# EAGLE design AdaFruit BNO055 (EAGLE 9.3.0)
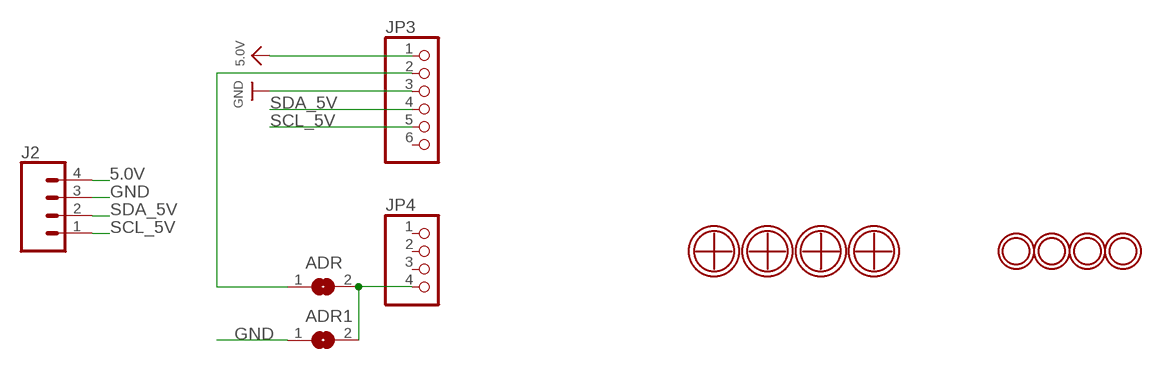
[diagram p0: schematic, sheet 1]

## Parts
ADR  SOLDERJUMPERREFLOW  [SOLDERJUMPER_REFLOW]
ADR1  SOLDERJUMPERREFLOW  [SOLDERJUMPER_REFLOW]
J2  CONN_04  [1X04]
JP3  HEADER-1X676MIL  [1X06_ROUND_76]
JP4  HEADER-1X476MIL  [1X04_ROUND_76]
U$1  3.2MM-5MM  [3.2MM-5MM]
U$3  3.2MM-5MM  [3.2MM-5MM]
U$4  3.2MM-5MM  [3.2MM-5MM]
U$5  3.2MM-5MM  [3.2MM-5MM]
U$7  MOUNTINGHOLE2.5_THICK  [MOUNTINGHOLE_2.5_PLATED_THICK]
U$8  MOUNTINGHOLE2.5_THICK  [MOUNTINGHOLE_2.5_PLATED_THICK]
U$9  MOUNTINGHOLE2.5_THICK  [MOUNTINGHOLE_2.5_PLATED_THICK]
U$11  MOUNTINGHOLE2.5_THICK  [MOUNTINGHOLE_2.5_PLATED_THICK]

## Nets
5.0V: J2.4 JP3.1
GND: ADR1.1 J2.3 JP3.3
N$1: ADR1.2 ADR.2 JP4.4
N$2: ADR.1 JP3.2
SCL_5V: J2.1 JP3.5
SDA_5V: J2.2 JP3.4
Unconnected: JP3.6 JP4.1 JP4.2 JP4.3 U$1.P$1 U$3.P$1 U$4.P$1 U$5.P$1

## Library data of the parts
ADR ADR1 = #microbuilder:SOLDERJUMPER: SMD Solder JUMPER
J2 = SparkFun-Connectors:CONN_04: Multi connection point. Often used as Generic Header-pin footprint for 0.1 inch spaced/style header connections On any of the 0.1 inch spaced packages, you can populate with these: Break Away Headers - Straight (PRT-00116) Break Away Male Headers - Right Angle (PRT-00553) Female Headers (PRT-00115)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; PROD_ID: CONN-09696
JP3 = microbuilder:HEADER-1X6: PIN HEADER
JP4 = microbuilder:HEADER-1X4: PIN HEADER
U$1 U$3-U$5 = #Holes:3.2MM-5MM
U$7-U$9 U$11 = microbuilder:MOUNTINGHOLE: Mounting Hole; BOM: EXCLUDE

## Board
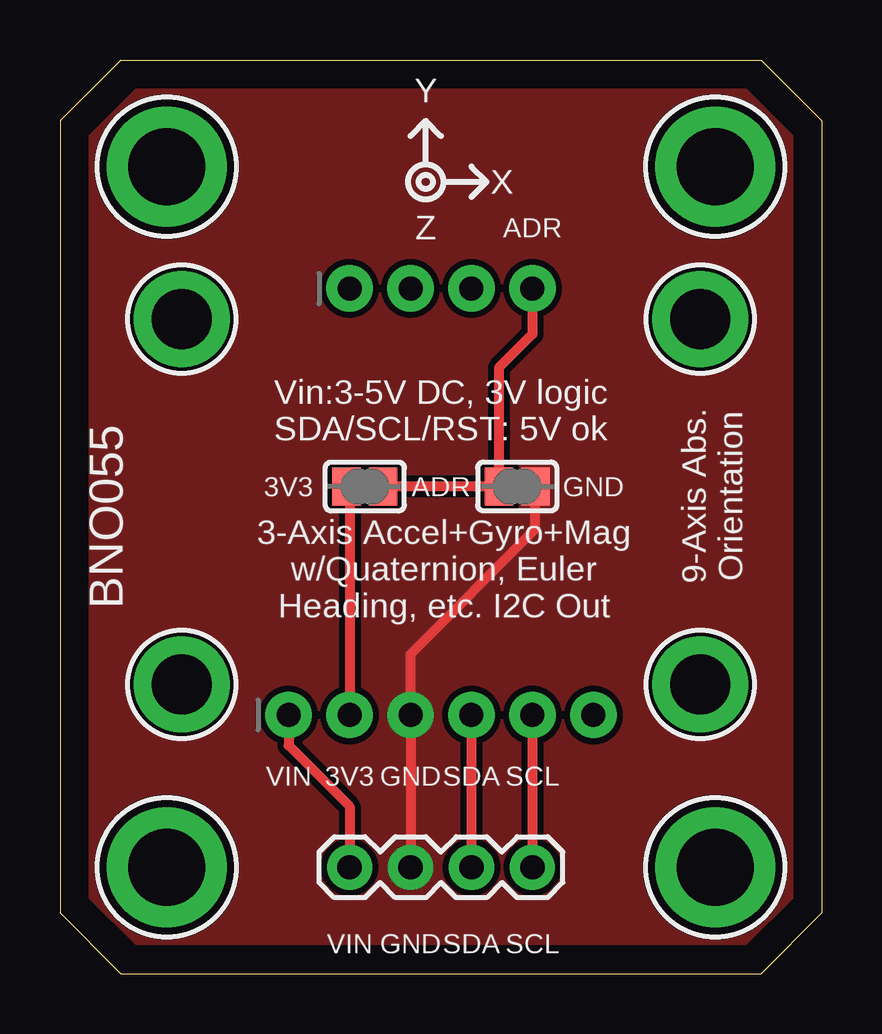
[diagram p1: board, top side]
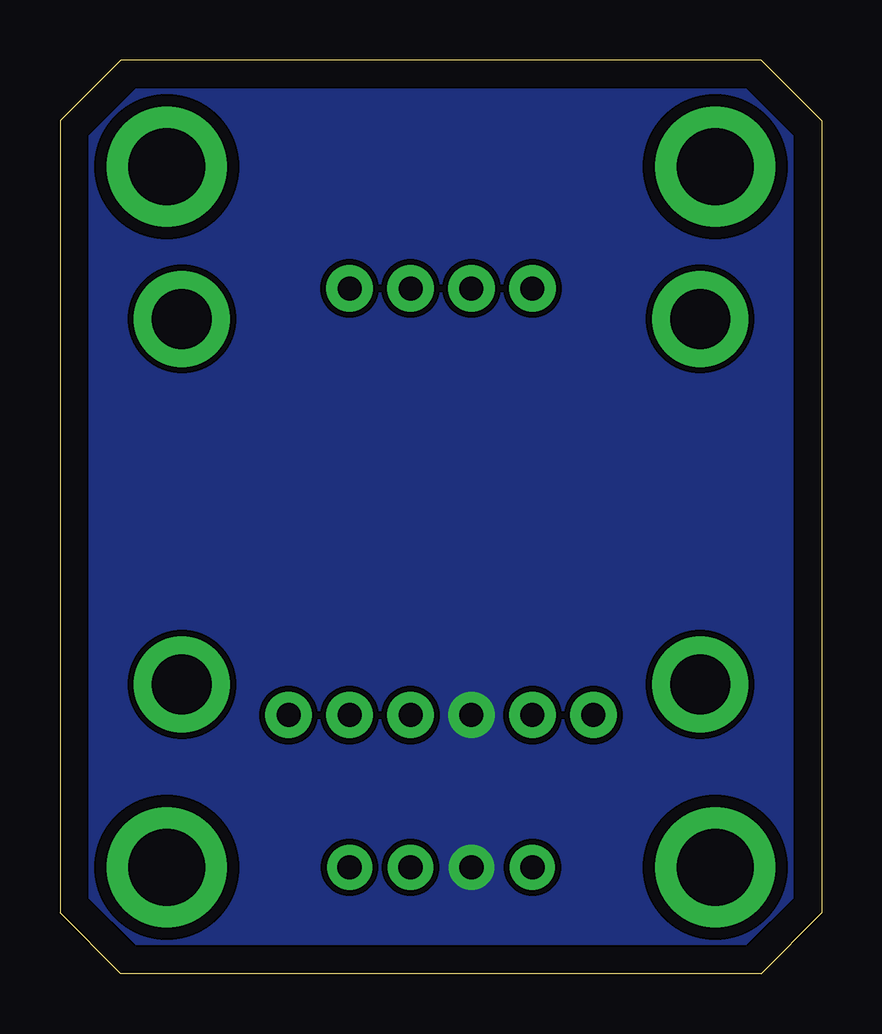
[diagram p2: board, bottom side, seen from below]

Size 31.75 x 38.1 mm. Coordinates in mm from the lower left corner, seen from the top.
Outline: 2.54,38.1 29.21,38.1 31.75,35.56 31.75,2.54 29.21,0 2.54,0 0,2.54 0,35.56 2.54,38.1
Copper layers (1*16): Top 0.035mm / dielectric 1.5mm / Bottom 0.035mm
Design rules "SparkFun 2 Layer Design Rule - STANDARD": minimum track width 10mil, minimum drill 20mil, track to track 10mil, track to pad 8mil, pad to pad 8mil, via to via 10mil, smd to smd 8mil, copper to edge 8mil, drill to drill 8mil, minimum pad ring 10mil, minimum via ring 10mil, stop-mask expansion 4mil, vias tented up to drill 25mil, thermal gap 10mil

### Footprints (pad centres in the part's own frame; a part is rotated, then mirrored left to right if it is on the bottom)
SOLDERJUMPER_REFLOW = smd 1.168 x 1.6: 1 -0.762,0; 2 0.762,0
1X04 = drill 1.016 pad 1.88: 1 0,0; 2 2.54,0; 3 5.08,0; 4 7.62,0
1X06_ROUND_76 = drill 1 pad 1.93: 1 -6.35,0; 2 -3.81,0; 3 -1.27,0; 4 1.27,0; 5 3.81,0; 6 6.35,0
1X04_ROUND_76 = drill 1 pad 1.93: 1 -3.81,0; 2 -1.27,0; 3 1.27,0; 4 3.81,0
3.2MM-5MM = drill 3.2 pad 5: P$1 0,0
MOUNTINGHOLE_2.5_PLATED_THICK = drill 2.5 pad 4: P$1 0,0

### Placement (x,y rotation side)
ADR  12.7,20.32 0 top
ADR1  19.05,20.32 180 top
J2  19.68,4.45 180 top
JP3  15.87,10.79 0 top
JP4  15.87,28.58 0 top
U$1  4.45,4.45 0 top
U$3  27.3,4.45 0 top
U$4  4.45,33.66 0 top
U$5  27.3,33.66 0 top
U$7  5.08,27.3 0 top
U$8  5.08,12.06 0 top
U$9  26.67,27.3 0 top
U$11  26.67,12.06 0 top

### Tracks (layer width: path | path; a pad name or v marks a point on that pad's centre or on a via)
5.0V
  Top 0.406: JP3.1 9.52,9.52 12.07,6.98 J2.4
GND
  Top 0.406: J2.3 JP3.3 14.6,13.34 19.81,18.54 ADR1.1
  pour Top (no thermals): 3.17,36.83 28.57,36.83 30.48,34.92 30.48,3.17 28.57,1.27 3.17,1.27 1.27,3.17 1.27,34.92
  pour Bottom (no thermals): 3.17,36.83 28.57,36.83 30.48,34.92 30.48,3.17 28.57,1.27 3.17,1.27 1.27,3.17 1.27,34.92
N$1
  Top 0.406: JP4.4 19.68,26.67 18.29,25.27 ADR1.2 ADR.2
N$2
  Top 0.406: ADR.1 12.07,20.19 JP3.2
SCL_5V
  Top 0.406: JP3.5 J2.1
SDA_5V
  Top 0.406: JP3.4 J2.2

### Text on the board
tPlace: Y | X | Z | ADR | Vin:3-5V DC, 3V logic / SDA/SCL/RST: 5V ok | 3V3 | GND | 9-Axis Abs. / Orientation | BNO055 | 3-Axis Accel+Gyro+Mag / w/Quaternion, Euler / Heading, etc. I2C Out | VIN | 3V3 | GND | SDA | SCL | VIN | GND | SDA | SCL

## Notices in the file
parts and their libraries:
SparkFun-Connectors: Licensing: Creative Commons ShareAlike 4.0 International - https://creativecommons.org/licenses/by-sa/4.0
microbuilder: This work is placed in the public domain, and may be freely used for commercial and non-commercial work with the following conditions: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
